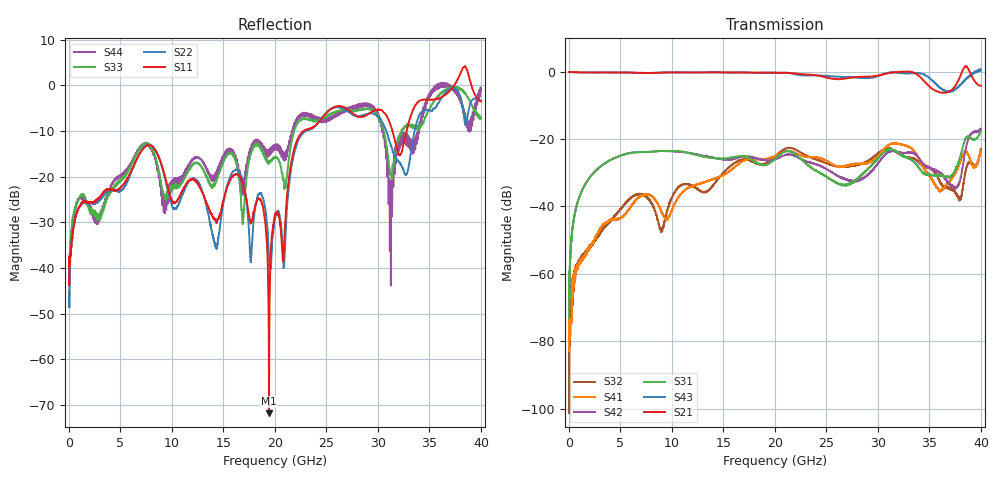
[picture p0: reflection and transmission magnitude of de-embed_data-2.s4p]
!Keysight Technologies,N5225B,MY51451420,A.15.40.08
!Date: Monday, July 18, 2022 07:52:52
!Correction: S11(C  4-Port  )
!S12(C  4-Port  )
!S13(C  4-Port  )
!S14(C  4-Port  )
!S21(C  4-Port  )
!S22(C  4-Port  )
!S23(C  4-Port  )
!S24(C  4-Port  )
!S31(C  4-Port  )
!S32(C  4-Port  )
!S33(C  4-Port  )
!S34(C  4-Port  )
!S41(C  4-Port  )
!S42(C  4-Port  )
!S43(C  4-Port  )
!S44(C  4-Port  )
!S4P File: Measurements: <S11,S12,S13,S14>,
!<S21,S22,S23,S24>,
!<S31,S32,S33,S34>,
!<S41,S42,S43,S44>:
# Hz S  dB  R 50
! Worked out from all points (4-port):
!   4000 points, 10 MHz to 40 GHz, reference 50 ohm
!   strongest paths, dB at 10 MHz, 10.01 GHz, 20.01 GHz, 30.01 GHz, 40 GHz:
!     S21: -0.1, -0.2, -0.3, -1.1, -4.2
!     S43: -0.1, -0.2, -0.3, -1.2, 0.4
!     S31: -59.5, -23.6, -25.9, -25.7, -17.7
!     S42: -69.7, -23.6, -26.0, -27.1, -17.0
!     S41: -70.7, -40.9, -25.0, -25.0, -23.6
!     S32: -60.3, -37.2, -25.1, -24.2, -23.0
!   lowest |S11| = -71.9 dB at 19.42 GHz (marker M1), VSWR 1.00, Z = 50 + j0.0131 ohm
!   |S11| at or under -10 dB: start of sweep to 22.76 GHz; 31.41 GHz to 32.78 GHz (1.37 GHz wide, 4.27 % of centre)
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1e7  -42.29 -144.5  -0.08 -0.4  -67.34 165.9  -64.75 11.3
     -0.07 -0.2  -46.32 129.0  -60.32 -141.5  -66.25 -117.3
     -59.46 37.4  -60.29 -67.2  -42.22 -147.2  -0.09 -0.1
     -70.66 -138.5  -69.68 -119.7  -0.10 -0.3  -47.14 6.2
9.51e9  -21.61 -86.9  -0.23 179.5  -23.50 -90.6  -43.90 49.7
        -0.22 179.5  -22.20 -92.1  -41.17 93.0  -23.58 -95.0
        -23.50 -90.5  -41.05 92.1  -23.79 -18.6  -0.18 175.4
        -43.78 50.5  -23.59 -95.1  -0.18 175.4  -23.28 -176.9
1.942e10  -71.87 149.1  -0.26 -20.4  -27.29 78.5  -25.66 -122.8
          -0.26 -20.6  -37.51 110.2  -26.66 -98.8  -26.34 59.3
          -27.33 78.4  -26.59 -98.7  -16.81 -49.0  -0.29 -29.1
          -25.67 -122.6  -26.31 59.5  -0.28 -29.2  -14.04 176.9
2.58e10  -4.71 -75.4  -2.17 -159.4  -32.67 -125.4  -27.85 85.9
         -2.16 -159.5  -4.86 -66.7  -27.94 109.5  -30.41 -147.8
         -32.62 -125.3  -27.96 109.4  -5.92 -65.0  -1.44 -169.2
         -27.86 85.9  -30.42 -148.0  -1.43 -169.3  -6.43 -102.0
3.107e10  -7.70 173.0  -0.39 78.1  -23.11 -2.0  -21.72 -13.9
          -0.39 77.9  -11.93 -164.8  -22.70 -0.2  -23.81 -3.2
          -23.09 -2.2  -22.73 -0.0  -17.75 -171.2  -0.27 68.2
          -21.70 -13.9  -23.84 -3.5  -0.25 68.1  -21.99 127.6
3.816e10  3.39 164.0  -0.08 -83.5  -23.23 -163.0  -25.31 -172.2
          -0.07 -83.8  -3.81 172.8  -36.03 -101.4  -29.27 -145.6
          -23.21 -162.9  -35.87 -101.1  -1.10 -173.4  -3.36 -96.5
          -25.39 -173.4  -29.21 -145.9  -3.35 -96.6  -4.81 173.0
4e10  -3.48 29.6  -4.16 -167.9  -17.71 105.3  -23.59 -48.6
      -4.17 -168.1  -3.41 -175.6  -23.01 36.9  -17.09 142.1
      -17.72 105.0  -22.97 36.9  -7.10 80.7  0.38 -145.4
      -23.60 -48.7  -17.04 142.4  0.40 -145.6  -1.08 101.4
